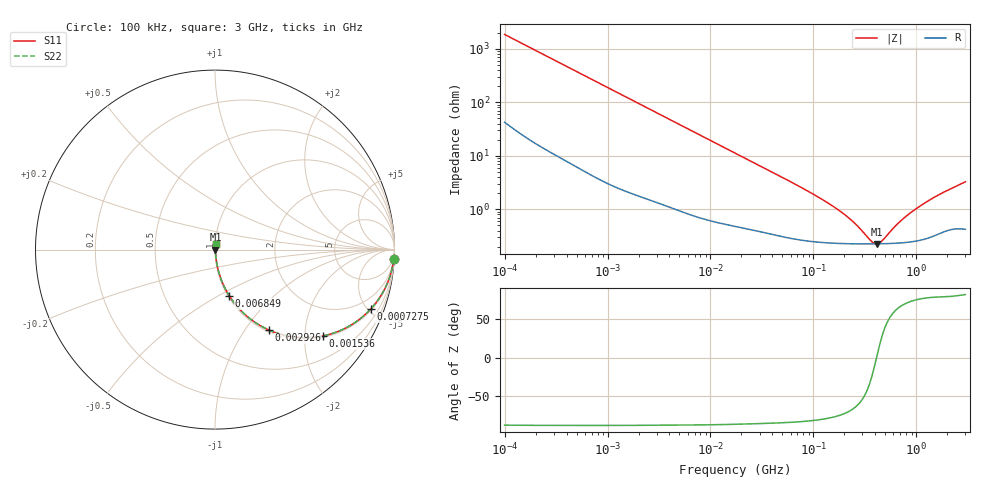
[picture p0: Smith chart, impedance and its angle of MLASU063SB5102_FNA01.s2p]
! MLASU063SB5102_FNA01  S-PARAMETER MODEL  ( Standard Model )
! Model Generated by TAIYO YUDEN Corporation (http://www.ty-top.com)
! Version 1.0
! TAIYO YUDEN Control No. 220601
! Copyright(c) 2012 TAIYO YUDEN CO.,LTD. All Rights Reserved.
! Product Description (link to TY-COMPAS)
! https://ds.yuden.co.jp/TYCOMPAS/or/detail?pn=MLASU063SB5102KFNA01&u=M
! Products Name : Multilayer Ceramic Capacitors
! Characteristics :
!  Capacitance : 1000 [pF] , Rated Voltage : 50 [V] , TCC : B / X5R
!  Case Size : 0.6 x 0.3 / 0.024 x 0.012 [mm/inch] , Thickness : 0.3 / 0.012 [mm/inch]
!  (Conditions: Temperature = 25 [degC] , DC Bias Voltage = 0 [V])
! External Node Assignments :
!  1  o---| |---o  2
! GND o---------o GND
! Frequency Range : 100kHz  -  3GHz  [ 401 STEP ]
# MHZ S RI R 50
! Freq[MHz].  S11 Real  S11 Imag  S21 Real  S21 Imag  S12 Real  S12 Imag  S22 Real  S22 Imag
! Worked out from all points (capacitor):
!   401 points, 100 kHz to 3 GHz, reference 50 ohm
!   read as one part in series: C = 857 pF near 105.3 kHz
!   lowest |Z| = 225 mohm at 412.4 MHz (marker M1)
!   series resonance near 411.2 MHz, so ESL is about 170 pH
!   S11 on the Smith chart (normalised r, x): 100 kHz: 2, -37; 727.5 kHz: 1.08, -5.18; 1.536 MHz: 1.04, -2.47; 2.926 MHz: 1.03, -1.30; 6.849 MHz: 1.02, -0.56; 3 GHz: 1.01, +0.06
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0.1  0.9959 -0.0537  0.00412 0.0537  0.00412 0.0537  0.9959 -0.0537
0.252895  0.9798 -0.1323  0.0202 0.1323  0.0202 0.1323  0.9798 -0.1323
0.562235  0.9143 -0.2719  0.0857 0.2719  0.0857 0.2719  0.9143 -0.2719
0.727522  0.8665 -0.3322  0.1335 0.3322  0.1335 0.3322  0.8665 -0.3322
1.043626  0.7629 -0.4173  0.2371 0.4173  0.2371 0.4173  0.7629 -0.4173
1.536162  0.6021 -0.4809  0.3979 0.4809  0.3979 0.4809  0.6021 -0.4809
2.925885  0.3023 -0.4489  0.6977 0.4489  0.6977 0.4489  0.3023 -0.4489
3.161081  0.2718 -0.4344  0.7282 0.4344  0.7282 0.4344  0.2718 -0.4344
4.534557  0.1576 -0.3528  0.8424 0.3528  0.8424 0.3528  0.1576 -0.3528
6.848882  0.0793 -0.2571  0.9207 0.2571  0.9207 0.2571  0.0793 -0.2571
17.7727  0.0164 -0.1072  0.9836 0.1072  0.9836 0.1072  0.0164 -0.1072
97.38194  0.00286 -0.0194  0.9971 0.0194  0.9971 0.0194  0.00286 -0.0194
200.3904  0.00233 -0.00764  0.9977 0.00764  0.9977 0.00764  0.00233 -0.00764
259.3015  0.00227 -0.00467  0.9977 0.00467  0.9977 0.00467  0.00227 -0.00467
362.5028  0.00224 -0.00124  0.9978 0.00124  0.9978 0.00124  0.00224 -0.00124
412.3589  0.00225 2.77e-05  0.9978 -2.77e-05  0.9978 -2.77e-05  0.00225 2.77e-05
457.1373  0.00226 0.00104  0.9977 -0.00104  0.9977 -0.00104  0.00226 0.00104
547.5153  0.00229 0.00284  0.9977 -0.00284  0.9977 -0.00284  0.00229 0.00284
745.9503  0.0024 0.00619  0.9976 -0.00619  0.9976 -0.00619  0.0024 0.00619
1097.999  0.00275 0.0113  0.9972 -0.0113  0.9972 -0.0113  0.00275 0.0113
1701.687  0.00387 0.0187  0.9961 -0.0187  0.9961 -0.0187  0.00387 0.0187
3000  0.00524 0.0321  0.9948 -0.0321  0.9948 -0.0321  0.00524 0.0321
